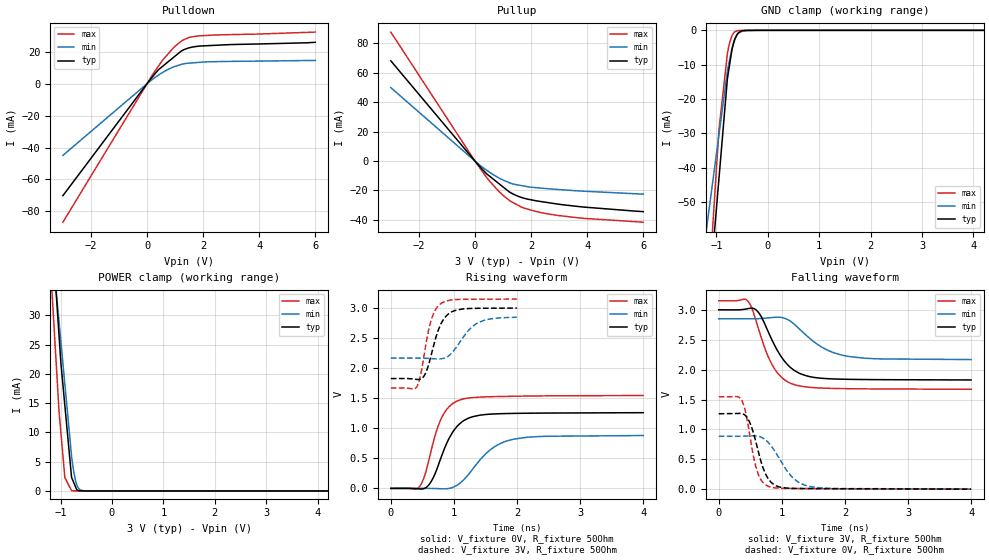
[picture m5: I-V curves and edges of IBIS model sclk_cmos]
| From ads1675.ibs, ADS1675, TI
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|   sclk_cmos Model
[Model]   sclk_cmos
Model_type   I/O
Polarity   Non-Inverting
Enable   Active-Low
Vinl = 0.9
Vinh = 2.1
Vmeas = 1.5
Vref = 0
Cref = 10pF
Rref = 500
|   typ   min   max
|   (nom PVT)   (Fast PVT)   (slow PVT)
|C_comp from frequency method(F=32MHz)
|Average
|C_comp   4.381e-12   4.309e-12   5.209e-12
|ON state : BUFFER OUTPUT TURNED HIGH
|C_comp   4.597e-12   4.506e-12   5.456e-12
|OFF state: BUFFER IN HIGH IMPEDANCE
C_comp   4.165e-12   4.111e-12   4.961e-12
|C_comp from L-C Tank method(L=1nH)
|ON state : BUFFER OUTPUT TURNED HIGH
|Resonant Frequency(Hz)   2.67e9   2.69e9   2.52e9
|C_comp   3.557e-12   3.504e-12   3.993e-12
|OFF state: BUFFER IN HIGH IMPEDANCE
|Resonant Frequency(Hz)   2.78e9   2.79e9   2.58e9
|C_comp   3.281e-12   3.257e-12   3.809e-12
| Where nom  PVT is Nominal Process,  3V,  51C
|   Fast PVT is Strong Process,   3.15V,  -40C
|   Slow PVT is Weak Process,   2.85V,  111C
[Model Spec]
Vinl   0.9   0.855   0.945
Vinh   2.1   1.995   2.205
[Voltage Range]   3   2.85   3.15
|Ambient Temperature   25   85   -40
|Junction Temperature
[Temperature Range]   51   111   -40
[Pullup Reference]   3   2.85   3.15
[Pulldown Reference]   0   0   0
[Power Clamp Reference]   3   2.85   3.15
[GND Clamp Reference]   0   0   0
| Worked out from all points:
|   slope of the pulldown table from 0 to 0.45 V, typ, clamps not added: 47.8 ohm
|   slope of the pullup table from 0 to 0.45 V, typ, clamps not added: 48.9 ohm
|   GND clamp passes 1 mA (typ) near -0.59 V on its own axis
|   POWER clamp passes 1 mA (typ) near -0.72 V on its own axis
|   falling waveform, V_fixture 3V, R_fixture 50Ohm: 20-80 % time 381ps typ, 527ps min, 335ps max; typ from 3 V to 1.83 V
|   rising waveform, V_fixture 0V, R_fixture 50Ohm: 20-80 % time 327ps typ, 475ps min, 273ps max; typ from 0 V to 1.26 V
|   rising waveform, V_fixture 3V, R_fixture 50Ohm: 20-80 % time 209ps typ, 311ps min, 170ps max; typ from 1.82 V to 3 V
|   falling waveform, V_fixture 0V, R_fixture 50Ohm: 20-80 % time 213ps typ, 348ps min, 171ps max; typ from 1.26 V to 0.002 V
[Pulldown]
|   Voltage   I(typ)   I(min)   I(max)
-3V       -70.2mA    -44.95mA   -86.83mA
153mV     3.489mA    2.2mA      4.415mA
420mV     8.976mA    5.561mA    11.37mA
554.4mV   10.9mA     7.047mA    14.73mA
913.5mV   16.06mA    10.29mA    22mA
1.093V    18.63mA    11.39mA    24.9mA
1.227V    20.56mA    12.15mA    26.64mA
1.515V    22.56mA    12.88mA    29.1mA
1.874V    23.59mA    13.42mA    30.01mA
6V        25.95mA    14.6mA     32.37mA
[GND Clamp]
|   Voltage   I(typ)   I(min)   I(max)
-3V       -1.064A    -972.5mA   -1.069A
-1.197V   -86.85mA   -58.32mA   -86.63mA
-951.3mV  -43.35mA   -30.58mA   -28.98mA
-786mV    -14.08mA   -11.92mA   -6.83mA
-759.1mV  -11.52mA   -9.76mA    -4.675mA
-737.1mV  -9.418mA   -8.118mA   -3.283mA
-693mV    -5.213mA   -5.288mA   -1.376mA
-642.6mV  -2.597mA   -2.766mA   -393.8uA
-601.4mV  -1.329mA   -1.395mA   -201.7uA
-570mV    -703.9uA   -766.4uA   -55.65uA
-478.8mV  -107.5uA   -116.2uA   -1.96uA
6V        0A         0A         0A
[Pullup]
|   Voltage   I(typ)   I(min)   I(max)
-3V       68.19mA    49.98mA    87.75mA
0V        0A         0A         0A
420mV     -8.738mA   -6.297mA   -11.24mA
554.4mV   -10.79mA   -8.014mA   -14.41mA
957.6mV   -16.93mA   -12.54mA   -22.56mA
1.269V    -21.5mA    -15.08mA   -27.35mA
1.764V    -25.39mA   -17.07mA   -32.1mA
2.57V     -28.19mA   -18.77mA   -35.86mA
3.934V    -31.4mA    -20.58mA   -39.06mA
6V        -34.42mA   -22.53mA   -41.61mA
[POWER Clamp]
|   Voltage   I(typ)   I(min)   I(max)
-3V       366mA      418.8mA    286.8mA
-1.208V   49.89mA    45.75mA    40.26mA
-1.033V   27.03mA    29.23mA    14.03mA
-993mV    21.79mA    25.44mA    9.915mA
-916.6mV  14.6mA     18.24mA    2.276mA
-784.3mV  2.279mA    5.769mA    19.85uA
-735.3mV  1.251mA    2.898mA    12.53uA
-712.5mV  772.8uA    1.926mA    9.134uA
-686.8mV  235.1uA    1.126mA    5.308uA
-635.5mV  45.83uA    310.1uA    109.3nA
-561.5mV  7.598uA    37.73uA    77.13nA
6V        0A         0A         0A
[Ramp]
R_load = 50
|   typ   min   max
dV/dt_r   0.754759/3.24891e-10   0.526984/4.73776e-10   0.926148/2.71931e-10
dV/dt_f   0.703497/3.81264e-10   0.408886/5.24098e-10   0.887018/3.34853e-10
[Falling Waveform]
V_fixture = 3V
V_fixture_min = 2.85V
V_fixture_max = 3.15V
R_fixture = 50Ohm
|   Time   V(typ)   V(min)   V(max)
0s        3V         2.85V      3.15V
461ps     3.019V     2.849V     3.148V
531ps     3.028V     2.85V      3.013V
627ps     2.96V      2.852V     2.692V
843ps     2.497V     2.871V     2.088V
983ps     2.228V     2.874V     1.884V
1.17ns    2.008V     2.783V     1.759V
1.607ns   1.858V     2.393V     1.693V
1.949ns   1.84V      2.244V     1.683V
3.999ns   1.828V     2.169V     1.672V
[Rising Waveform]
V_fixture = 0V
V_fixture_min = 0V
V_fixture_max = 0V
R_fixture = 50Ohm
|   Time   V(typ)   V(min)   V(max)
0s        1.886nV    2.462nV    1.56nV
455ps     -8.956mV   480.2uV    28.73mV
546ps     5.746mV    362.9uV    243.3mV
630ps     98.15mV    -400.1uV   590.5mV
793ps     504.5mV    -6.327mV   1.147V
923ps     831.6mV    -1.427mV   1.357V
1.073ns   1.056V     69.14mV    1.462V
1.511ns   1.229V     582.4mV    1.521V
1.849ns   1.244V     792.1mV    1.529V
3.999ns   1.258V     878.3mV    1.544V
[Rising Waveform]
V_fixture = 3V
V_fixture_min = 2.85V
V_fixture_max = 3.15V
R_fixture = 50Ohm
|   Time   V(typ)   V(min)   V(max)
0s        1.825V     2.164V     1.669V
412ps     1.81V      2.165V     1.688V
459ps     1.812V     2.165V     1.826V
526ps     1.866V     2.163V     2.205V
630ps     2.175V     2.158V     2.763V
690ps     2.418V     2.154V     2.934V
798ps     2.743V     2.153V     3.075V
974ps     2.938V     2.259V     3.133V
1.359ns   2.992V     2.739V     3.143V
1.997ns   2.996V     2.843V     3.146V
[Falling Waveform]
V_fixture = 0V
V_fixture_min = 0V
V_fixture_max = 0V
R_fixture = 50Ohm
|   Time   V(typ)   V(min)   V(max)
0s        1.262V     886.5mV    1.546V
361ps     1.266V     887.2mV    1.492V
417ps     1.239V     888.9mV    1.326V
488ps     1.125V     892.2mV    931.2mV
606ps     718.8mV    889.4mV    315.2mV
704ps     352.6mV    854.1mV    110.4mV
797ps     156.9mV    768.6mV    44.37mV
1.16ns    15.77mV    207.7mV    13.77mV
1.453ns   11.66mV    43.67mV    11.79mV
3.999ns   2.422mV    4.501mV    2.099mV
